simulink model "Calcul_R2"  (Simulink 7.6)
settings: Solver=ode45  StartTime=0.0  StopTime=10.0  RelTol=1e-3
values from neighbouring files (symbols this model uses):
  R = 1e3    (= 1000)    [oscillateur_dephasage.m]    (also in Calcul_Ampl_phase_A.m = 1; circuit_RLC_parallele_.m = 4; symbolique_circuit_RC.m = 4; parametres.m = 4)
libraries: fl_lib x13, nesl_utility x3, elec_lib x1

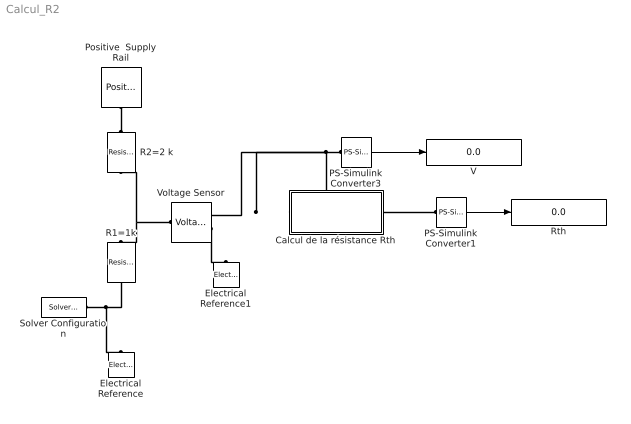
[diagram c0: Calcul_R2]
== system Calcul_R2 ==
  Calcul de la résistance Rth : Subsystem
  Electrical Reference : fl_lib/Electrical/Electrical Elements/Electrical Reference  DialogController=NetworkEngine.DynNeDlgSource  SystemSampleTime=-1  i_Log=off  LocalVarNames=|i  LocalVarDescs=|i  LocalVarLogging=[]
  Electrical Reference1 : fl_lib/Electrical/Electrical Elements/Electrical Reference  DialogController=NetworkEngine.DynNeDlgSource  SystemSampleTime=-1  i_Log=off  LocalVarNames=|i  LocalVarDescs=|i  LocalVarLogging=[]
  PS-Simulink Converter1 : nesl_utility/PS-Simulink Converter  DialogController=NetworkEngine.DynNeUtilDlgSource  SystemSampleTime=-1  PhysicalDomain=network_engine_domain  LeftPortType=input  RightPortType=output  SubClassName=ps_output  Unit=V  AffineConversion=off
  PS-Simulink Converter3 : nesl_utility/PS-Simulink Converter  DialogController=NetworkEngine.DynNeUtilDlgSource  SystemSampleTime=-1  PhysicalDomain=network_engine_domain  LeftPortType=input  RightPortType=output  SubClassName=ps_output  Unit=V  AffineConversion=off
  Positive  Supply Rail : elec_lib/Sources/Positive Supply Rail  DialogController=NetworkEngine.DynNeDlgSource  SystemSampleTime=-1  v0=Vcc V  current_Log=off  voltage_Log=off  power_Log=off  LocalVarNames=|current|voltage|power  LocalVarDescs=|Current (A)|Voltage (V)|Power (W)  LocalVarLogging=[0 0 0]
  R1=1k : fl_lib/Electrical/Electrical Elements/Resistor  DialogController=NetworkEngine.DynNeDlgSource  SystemSampleTime=-1  R=R Ohm  i_Log=off  v_Log=off  LocalVarNames=|current|voltage|power  LocalVarDescs=|Resistor current (A)|Voltage across resistor (V)|Power (W)  LocalVarLogging=[0 0 0]
  R2=2 k : fl_lib/Electrical/Electrical Elements/Resistor  DialogController=NetworkEngine.DynNeDlgSource  SystemSampleTime=-1  R=2*R Ohm  i_Log=off  v_Log=off  LocalVarNames=|current|voltage|power  LocalVarDescs=|Resistor current (A)|Voltage across resistor (V)|Power (W)  LocalVarLogging=[0 0 0]
  Rth : Display
  Solver Configuration : nesl_utility/Solver Configuration  DialogController=NetworkEngine.DynNeUtilDlgSource  SystemSampleTime=-1  PhysicalDomain=network_engine_domain  LeftPortType=input  RightPortType=generic  SubClassName=solver  Accelerate=off  Profile=off  ResidualTolerance=1e-9  MaxNonlinIter=12  MaxModeIter=2  DoFixedCost=off  UseLocalSampling=off  DoDC=off  LinearAlgebra=Sparse  LocalSolverSampleTime=.001  LocalSolverChoice=NE_BACKWARD_EULER_ADVANCER  UseLocalSolver=off
  V : Display
  Voltage Sensor : fl_lib/Electrical/Electrical Sensors/Voltage Sensor  DialogController=NetworkEngine.DynNeDlgSource  SystemSampleTime=-1  i1_Log=off  v1_Log=off  LocalVarNames=|i1|v1  LocalVarDescs=|i1|v1  LocalVarLogging=[]
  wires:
  PS-Simulink Converter1/1 -> Rth/1
  PS-Simulink Converter3/1 -> V/1
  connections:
  Voltage Sensor/LConn1 -- R1=1k/RConn1 -- R2=2 k/LConn1
  Solver Configuration/RConn1 -- R1=1k/LConn1 -- Electrical Reference/LConn1
  PS-Simulink Converter3/LConn1 -- Voltage Sensor/RConn1 -- Calcul de la résistance Rth/LConn1
  Calcul de la résistance Rth/RConn1 -- PS-Simulink Converter1/LConn1
  R2=2 k/RConn1 -- Positive  Supply Rail/RConn1
  Voltage Sensor/RConn2 -- Electrical Reference1/LConn1

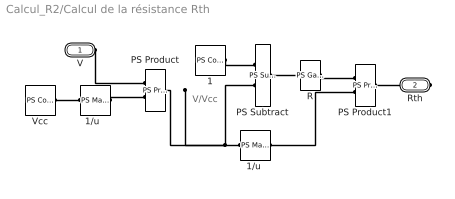
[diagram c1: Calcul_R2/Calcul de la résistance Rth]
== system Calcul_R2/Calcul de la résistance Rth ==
  note: V/Vcc
  1 : fl_lib/Physical Signals/Sources/PS Constant  DialogController=NetworkEngine.DynNeDlgSource  SystemSampleTime=-1  constant=1  LocalVarLogging=[]
  "1/u " : fl_lib/Physical Signals/Functions/PS Math Function  DialogController=NetworkEngine.DynNeDlgSource  SystemSampleTime=-1  fcn_choice=9  LocalVarLogging=[]
  "1/u  " : fl_lib/Physical Signals/Functions/PS Math Function  DialogController=NetworkEngine.DynNeDlgSource  SystemSampleTime=-1  fcn_choice=9  LocalVarLogging=[]
  PS Product : fl_lib/Physical Signals/Functions/PS Product  DialogController=NetworkEngine.DynNeDlgSource  SystemSampleTime=-1  LocalVarLogging=[]
  PS Product1 : fl_lib/Physical Signals/Functions/PS Product  DialogController=NetworkEngine.DynNeDlgSource  SystemSampleTime=-1  LocalVarLogging=[]
  PS Subtract : fl_lib/Physical Signals/Functions/PS Subtract  DialogController=NetworkEngine.DynNeDlgSource  SystemSampleTime=-1  LocalVarLogging=[]
  R : fl_lib/Physical Signals/Functions/PS Gain  DialogController=NetworkEngine.DynNeDlgSource  SystemSampleTime=-1  gain=R  LocalVarLogging=[]
  Vcc : fl_lib/Physical Signals/Sources/PS Constant  DialogController=NetworkEngine.DynNeDlgSource  SystemSampleTime=-1  constant=Vcc  LocalVarLogging=[]
  V : PMIOPort  Port=1  Side=Left
  Rth : PMIOPort  Port=2  Side=Right
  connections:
  1/RConn1 -- PS Subtract/LConn1
  Vcc/RConn1 -- "1/u  "/LConn1
  "1/u  "/RConn1 -- PS Product/LConn2
  "1/u "/LConn1 -- PS Subtract/LConn2 -- PS Product/RConn1
  "1/u "/RConn1 -- PS Product1/LConn2
  R/RConn1 -- PS Product1/LConn1
  PS Subtract/RConn1 -- R/LConn1
  V/RConn1 -- PS Product/LConn1
  Rth/RConn1 -- PS Product1/RConn1
